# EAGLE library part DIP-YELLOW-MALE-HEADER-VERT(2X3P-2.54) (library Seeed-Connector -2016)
320020027
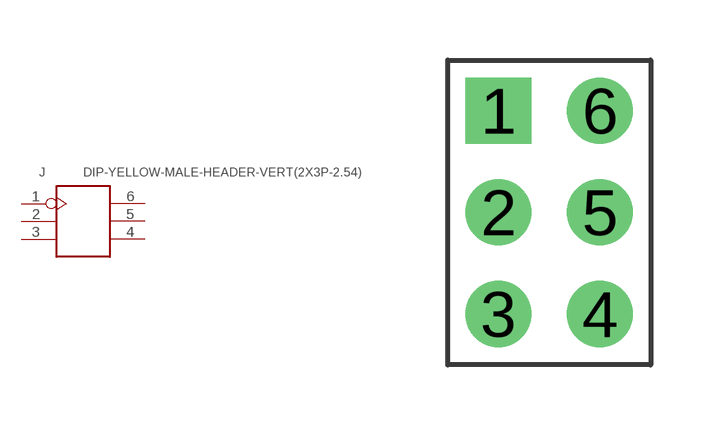
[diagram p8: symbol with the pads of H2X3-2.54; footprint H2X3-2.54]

Designator prefix J

## DIP-YELLOW-MALE-HEADER-VERT(2X3P-2.54) (MPN: P125-1203A0BS116A2; VALUE: YELLOW-2X3P-2.54)  [H2X3-2.54]
1  1
2  2
3  3
4  4
5  5
6  6

## Footprint H2X3-2.54 (pad centres in mm)
drill 0.889 pad 1.651 square: 1 -1.27,2.54
drill 0.889 pad 1.651: 2 -1.27,0; 3 -1.27,-2.54; 4 1.27,-2.54; 5 1.27,0; 6 1.27,2.54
